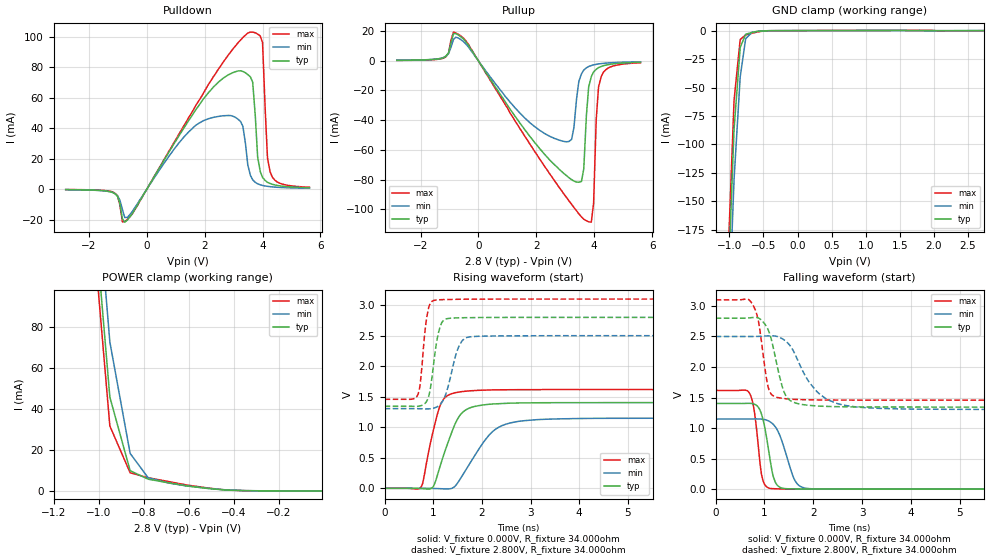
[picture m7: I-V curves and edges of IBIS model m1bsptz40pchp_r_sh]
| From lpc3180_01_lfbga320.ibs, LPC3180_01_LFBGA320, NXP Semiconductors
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| |   Rev 0.20 IBIS Model Design Automation Generation   |
| |   N O N - S I L I C O N   C O R R E L A T E D   |
| |   This IBIS [Model] is pre-Beta tactical support   |
| |  Note: this IBIS [Model] contains clamp curves generated   |
| |   through simulation which should not be relied upon   |
| mem1bsptz40pchp
|   Bidirectional Pad 2.8
|   3state Output
|   Plain Input
|   1ns Slew Rate control
|   CMOS
| Repeater Mode (p1=1, p2=0)
[Model]   m1bsptz40pchp_r_sh | of mem1bsptz40pchp
Model_type   I/O
Polarity   Non-Inverting
Enable   Active-Low
|  Reciever Thresholds
Vinl   = 0.36V
Vinh   = 0.84V
| AC Test Load Conditions
Vref   = 0
Cref   = 1.2e-11
Rref   = 1000000000
Vmeas   = 0.6
| [Process Range]   typical   min   max
| C_comp edge width   400.000ps   400.000ps   400.000ps
| C_comp Tstrobe   40.000fs   40.000fs   40.000fs
C_comp   2.018pF   1.943pF   2.108pF
[Temperature Range]   25   125   -40
[Voltage Range]   2.80V   2.50V   3.10V
[GND Clamp Reference]   0.00V   0.00V   0.00V
[Pulldown Reference]   0.00V   0.00V   0.00V
[POWER Clamp Reference]   2.80V   2.50V   3.10V
[Pullup Reference]   2.80V   2.50V   3.10V
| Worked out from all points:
|   slope of the pulldown table from 0 to 0.42 V, typ, clamps not added: 31 ohm
|   slope of the pullup table from 0 to 0.42 V, typ, clamps not added: 32.9 ohm
|   GND clamp passes 1 mA (typ) near -0.61 V on its own axis
|   POWER clamp passes 1 mA (typ) near -0.49 V on its own axis
|   rising waveform, V_fixture 0.000V, R_fixture 34.000ohm: 20-80 % time 382ps typ, 592ps min, 274ps max; typ from 0 V to 1.4 V
|   falling waveform, V_fixture 0.000V, R_fixture 34.000ohm: 20-80 % time 183ps typ, 282ps min, 135ps max; typ from 1.4 V to 0 V
|   rising waveform, V_fixture 2.800V, R_fixture 34.000ohm: 20-80 % time 156ps typ, 236ps min, 119ps max; typ from 1.34 V to 2.8 V
|   falling waveform, V_fixture 2.800V, R_fixture 34.000ohm: 20-80 % time 261ps typ, 557ps min, 175ps max; typ from 2.8 V to 1.34 V
[GND Clamp]
| ref voltage   0.00V   0.00V   0.00V
|   Voltage   I(typ)   I(min)   I(max)
-2.8V     -3.643A    -3.653A    -3.644A
-1.01V    -211.8mA   -255.9mA   -186.6mA
-930mV    -86.6mA    -130.6mA   -61.24mA
-840mV    -14.83mA   -40.64mA   -7.829mA
-760mV    -3.203mA   -7.088mA   -3.83mA
-670mV    -1.622mA   -1.69mA    -2.382mA
-500mV    -233.9uA   -204.7uA   -414uA
2.73V     -11.67uA   31.94uA    -74.22uA
[Power Clamp]   | Vtable = Vcc - Vpad
| ref voltage   2.80V   2.50V   3.10V
|   Voltage   I(typ)   I(min)   I(max)
-2.82V    3.531A     3.518A     3.546A
-1.03V    149.7mA    178.4mA    134.4mA
-950mV    45.72mA    72.62mA    31.66mA
-860mV    9.875mA    18.31mA    8.866mA
-780mV    5.725mA    6.415mA    6.434mA
-690mV    3.961mA    3.875mA    4.58mA
-610mV    2.472mA    2.439mA    2.908mA
-440mV    442.3uA    569.4uA    500uA
-270mV    46.38uA    47.88uA    58.33uA
-10mV     1.584uA    1.118uA    2.104uA
[Pulldown]
| ref voltage   0.00V   0.00V   0.00V
|   Voltage   I(typ)   I(min)   I(max)
-2.8V     -319.3uA   -345.4uA   -253.1uA
-1.18V    -2.159mA   -2.186mA   -1.786mA
-670mV    -20.28mA   -18.52mA   -19.91mA
2.13V     63.32mA    46.22mA    68.69mA
3.24V     77.68mA    44.42mA    97.81mA
3.58V     73.7mA     9.097mA    103.1mA
3.66V     70.11mA    6.079mA    103.1mA
3.83V     21.16mA    3.502mA    101.8mA
4V        7.734mA    2.421mA    96.19mA
4.17V     4.509mA    1.835mA    20.55mA
4.26V     3.717mA    1.634mA    11.45mA
5.62V     949.5uA    582uA      1.271mA
[Pullup]   | Vtable = Vcc - Vpad
| ref voltage   2.80V   2.50V   3.10V
|   Voltage   I(typ)   I(min)   I(max)
-2.82V    285.4uA    305.9uA    228.1uA
-520mV    14.74mA    12.98mA    15.34mA
2.79V     -73.12mA   -53.48mA   -85.35mA
3.22V     -80.05mA   -52.98mA   -96.69mA
3.47V     -81.85mA   -13.92mA   -103.2mA
3.64V     -72.85mA   -6.25mA    -106.7mA
3.81V     -17.56mA   -3.872mA   -108.5mA
3.9V      -10.74mA   -3.234mA   -108.8mA
3.98V     -7.509mA   -2.77mA    -95.89mA
4.07V     -5.754mA   -2.418mA   -39.51mA
4.24V     -3.885mA   -1.924mA   -10.84mA
5.6V      -1.045mA   -712.7uA   -1.375mA
[Ramp]
R_load   = 34.000ohm
|   dV/dt(typ)   dV/dt(min)   dV/dt(max)
dV/dt_r   972.504mV/345.000ps   809.695mV/540.000ps   1.111V/250.000ps
dV/dt_f   1.002V/240.000ps   841.229mV/475.000ps   1.124V/165.000ps
[Rising Waveform]  | cubic spline decimation from 2001 points
V_fixture   = 0.000V
R_fixture   = 34.000ohm
|   Time   V(typ)   V(min)   V(max)
0s        4.292nV    139.7nV    2.459nV
750ps     -4.658mV   315.5uV    23.5mV
995ps     24.02mV    -2.306mV   924.1mV
1.13ns    332.7mV    -5.781mV   1.332V
1.25ns    630.1mV    -10.44mV   1.493V
1.465ns   1.081V     49.96mV    1.568V
1.695ns   1.296V     333.9mV    1.593V
2.16ns    1.377V     882.3mV    1.611V
2.755ns   1.398V     1.097V     1.616V
10ns      1.404V     1.148V     1.617V
[Falling Waveform]  | cubic spline decimation from 2001 points
V_fixture   = 0.000V
R_fixture   = 34.000ohm
|   Time   V(typ)   V(min)   V(max)
0s        1.404V     1.148V     1.617V
705ps     1.405V     1.148V     1.554V
795ps     1.391V     1.149V     1.261V
940ps     1.226V     1.148V     240.9mV
1.11ns    509mV      1.105V     13.37mV
1.185ns   192.8mV    1.057V     7.983mV
1.28ns    51.33mV    942.1mV    4.991mV
1.615ns   3.647mV    154.8mV    1.649mV
1.85ns    1.805mV    14.65mV    894.6uV
10ns      150.6nV    560.3uV    80.96nV
[Rising Waveform]  | cubic spline decimation from 2001 points
V_fixture   = 2.800V
V_fixture_min = 2.500V
V_fixture_max = 3.100V
R_fixture   = 34.000ohm
|   Time   V(typ)   V(min)   V(max)
0s        1.344V     1.305V     1.458V
685ps     1.344V     1.305V     1.534V
735ps     1.351V     1.304V     1.733V
830ps     1.39V      1.301V     2.572V
890ps     1.467V     1.301V     2.904V
1.045ns   2.27V      1.323V     3.083V
1.215ns   2.754V     1.458V     3.092V
1.53ns    2.793V     2.332V     3.097V
1.75ns    2.795V     2.481V     3.098V
10ns      2.8V       2.5V       3.1V
[Falling Waveform]  | cubic spline decimation from 2001 points
V_fixture   = 2.800V
V_fixture_min = 2.500V
V_fixture_max = 3.100V
R_fixture   = 34.000ohm
|   Time   V(typ)   V(min)   V(max)
0s        2.8V       2.5V       3.1V
735ps     2.809V     2.5V       3.053V
870ps     2.805V     2.502V     2.774V
1.085ns   2.591V     2.51V      1.645V
1.305ns   1.857V     2.488V     1.495V
1.42ns    1.557V     2.433V     1.482V
1.575ns   1.429V     2.288V     1.472V
2.065ns   1.363V     1.605V     1.462V
2.695ns   1.349V     1.366V     1.459V
10ns      1.344V     1.305V     1.458V
